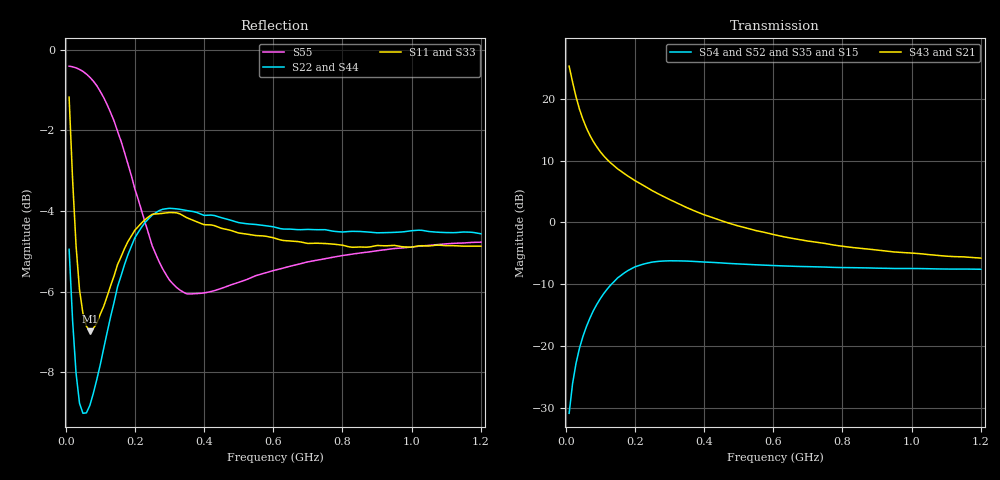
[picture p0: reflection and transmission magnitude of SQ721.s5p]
!  POLYFET RF DEVICES
!  S PARAMETERS FOR
!  SQ721 (EACH SIDE)
!  VDS=12.5, IDQ=200MA
!AWR Design Environment (2053) Wed Feb 04 15:38:15 2004
!freq-unit  param-type  data-format  keyword  impedance-ohms
# MHz  S  MA  R  50
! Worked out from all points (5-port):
!   120 points, 10 MHz to 1.2 GHz, reference 50 ohm
!   strongest paths, dB at 10 MHz, 310 MHz, 610 MHz, 910 MHz, 1.2 GHz:
!     S43: 25.3, 3.5, -2.1, -4.5, -5.8
!     S21: 25.3, 3.5, -2.1, -4.5, -5.8
!     S54: -30.9, -6.2, -7.0, -7.4, -7.6
!     S52: -30.9, -6.2, -7.0, -7.4, -7.6
!     S35: -32.9, -6.4, -7.2, -7.6, -7.8
!     S15: -32.9, -6.4, -7.2, -7.6, -7.8
!   lowest |S11| = -7.0 dB at 70 MHz (marker M1), VSWR 2.62, Z = 45.9 - j47.8 ohm
!   |S11| at or under -10 dB: nowhere
